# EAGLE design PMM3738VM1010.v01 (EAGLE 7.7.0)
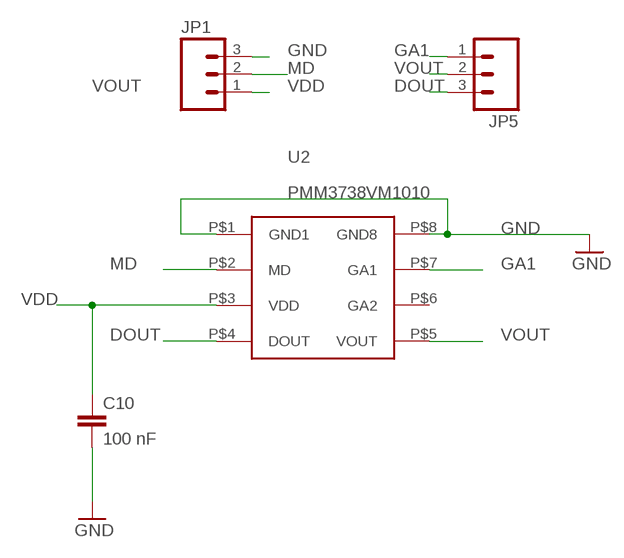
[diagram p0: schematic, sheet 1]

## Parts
C10  100 nF  0402CAP.KW  [0402-CAP]
JP1  M031X03_NO_SILK  [1X03_NO_SILK]
JP5  M031X03_NO_SILK  [1X03_NO_SILK]
U2  PMM3738VM1010  [PMM3738VM1010]

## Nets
DOUT: JP5.3 U2.P$4(DOUT)
GA1: JP5.1 U2.P$7(GA1)
GND: C10.2 JP1.3 U2.P$1(GND1) U2.P$8(GND8)
MD: JP1.2 U2.P$2(MD)
VDD: C10.1 JP1.1 U2.P$3(VDD)
VOUT: JP5.2 U2.P$5(VOUT)
Unconnected: U2.P$6(GA2)

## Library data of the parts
C10 = SparkFun-Capacitors:0402CAP.KW
JP1 JP5 = SparkFun-Connectors:M03: Header 3 Standard 3-pin 0.1" header. Use with straight break away headers (SKU : PRT-00116), right angle break away headers (PRT-00553), swiss pins (PRT-00743), machine pins (PRT-00117), and female headers (PRT-00115). Molex polarized connector foot print use with SKU : PRT-08232 with associated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
U2 = kris:PMM3738VM1010: PUI Audio's VESPER PMM-3738-VM1010-R Wake-on-Sound Analog Microphone

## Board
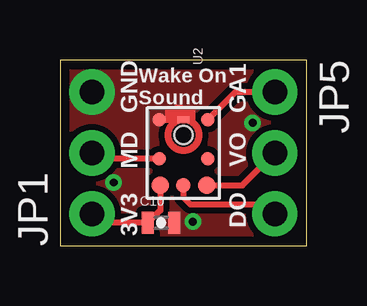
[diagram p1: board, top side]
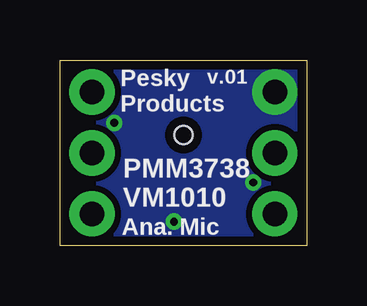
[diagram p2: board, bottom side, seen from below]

Size 10.29 x 7.75 mm. Coordinates in mm from the lower left corner, seen from the top.
Outline: 0,0 10.29,0 10.29,7.75 0,7.75 0,0
Copper layers (1*16): Top 0.0356mm / dielectric 1.5011mm / Bottom 0.0356mm
Design rules "LaenPCBOrder *": minimum track width 6mil, minimum drill 13mil, track to track 6mil, track to pad 6mil, pad to pad 6mil, via to via 6mil, smd to smd 6mil, copper to edge 15mil, drill to drill 6mil, minimum pad ring 7mil, minimum via ring 7mil, stop-mask expansion 3mil, vias tented up to drill 20mil, thermal gap 10mil

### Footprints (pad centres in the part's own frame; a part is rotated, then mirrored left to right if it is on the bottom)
0402-CAP = smd 0.5 x 0.9: 1 -0.55,0; 2 0.55,0
1X03_NO_SILK = drill 1.016 pad 1.88: 1 0,0; 2 2.54,0; 3 5.08,0
PMM3738VM1010 = smd 0.562 x 0.562: P$1 -1.39,-1.015; P$2 0.25,-1.015; P$6 0.25,1.015; P$7 -1.39,1.015 | smd 0.723 x 0.723: P$3 1.35,-0.965; P$5 1.35,0.965 | smd 0.612 x 0.612: P$4 1.35,0 | smd 0.3 x 0.5: P$8 -1.38,0 | hole 0.75: -0.75,0

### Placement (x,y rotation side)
C10  4.22,0.97 0 top
JP1  1.33,1.33 90 top
JP5  8.95,6.41 270 top
U2  5.14,3.87 270 top

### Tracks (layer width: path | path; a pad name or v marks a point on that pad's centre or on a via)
DOUT
  Top 0.254: U2.P$4 5.14,2.02 5.44,1.73 8.56,1.73 JP5.3
GA1
  Top 0.254: JP5.1 7.31,6.41 U2.P$7
GND  (via drill 0.33)
  Top 0.305: U2.P$8 5.46,5.25 5.49,5.28 5.49,5.69 5.18,5.69 5.18,5.28 5.03,5.28 5.03,5.74 4.88,5.74 4.83,5.69 4.83,5.28 4.72,5.28 4.72,5.64 4.57,5.64 4.52,5.59 4.52,5.44 4.67,5.28 4.15,5.28 U2.P$1
  Top 0.406: U2.P$1
  other vias: 5.54,1.02 2.24,2.64 8.03,5.13
  pour Bottom (isolate 0.254, no thermals): 0,7.75 10.29,7.75 10.29,0 0,0
  pour Top (isolate 0.254, no thermals): 0,7.75 10.29,7.75 10.29,0 0,0
MD
  Top 0.254: U2.P$2 1.58,3.62 JP1.2
VDD
  Top 0.254: U2.P$3 4.18,1.48 C10.1 1.7,0.96 JP1.1
VOUT
  Top 0.254: U2.P$5 7.6,2.52 JP5.2

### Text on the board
tPlace: GND | Wake On / Sound | GA1 | MD | VO | DO | 3V3
bPlace: v.01 | Pesky / Products | PMM3738 / VM1010 | Ana. Mic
